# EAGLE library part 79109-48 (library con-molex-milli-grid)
RECEPTACAL
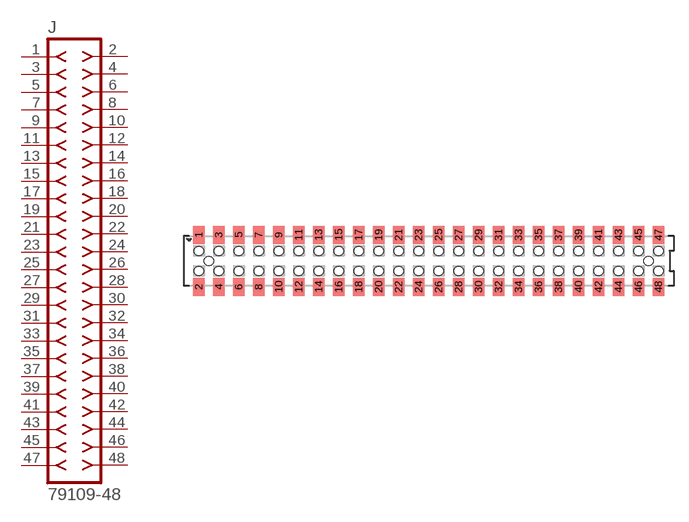
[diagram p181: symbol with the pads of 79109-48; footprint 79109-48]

Designator prefix J

## 79109-48  [79109-48]
1  1  pas
2  2  pas
3  3  pas
4  4  pas
5  5  pas
6  6  pas
7  7  pas
8  8  pas
9  9  pas
10  10  pas
11  11  pas
12  12  pas
13  13  pas
14  14  pas
15  15  pas
16  16  pas
17  17  pas
18  18  pas
19  19  pas
20  20  pas
21  21  pas
22  22  pas
23  23  pas
24  24  pas
25  25  pas
26  26  pas
27  27  pas
28  28  pas
29  29  pas
30  30  pas
31  31  pas
32  32  pas
33  33  pas
34  34  pas
35  35  pas
36  36  pas
37  37  pas
38  38  pas
39  39  pas
40  40  pas
41  41  pas
42  42  pas
43  43  pas
44  44  pas
45  45  pas
46  46  pas
47  47  pas
48  48  pas

## Footprint 79109-48 (pad centres in mm)
RECEPTACAL SMD Dual Row, Vertical, Pass-Thru
smd 1.12 x 1.83: 1 -23,2.6; 2 -23,-2.6; 3 -21,2.6; 4 -21,-2.6; 5 -19,2.6; 6 -19,-2.6; 7 -17,2.6; 8 -17,-2.6; 9 -15,2.6; 10 -15,-2.6; 11 -13,2.6; 12 -13,-2.6; 13 -11,2.6; 14 -11,-2.6; 15 -9,2.6; 16 -9,-2.6; 17 -7,2.6; 18 -7,-2.6; 19 -5,2.6; 20 -5,-2.6; 21 -3,2.6; 22 -3,-2.6; 23 -1,2.6; 24 -1,-2.6; 25 1,2.6; 26 1,-2.6; 27 3,2.6; 28 3,-2.6; 29 5,2.6; 30 5,-2.6; 31 7,2.6; 32 7,-2.6; 33 9,2.6; 34 9,-2.6; 35 11,2.6; 36 11,-2.6; 37 13,2.6; 38 13,-2.6; 39 15,2.6; 40 15,-2.6; 41 17,2.6; 42 17,-2.6; 43 19,2.6; 44 19,-2.6; 45 21,2.6; 46 21,-2.6; 47 23,2.6; 48 23,-2.6
hole 0.914 at -22,0
hole 0.914 at -23,1
hole 0.914 at -23,-1
hole 0.914 at -21,-1
hole 0.914 at -21,1
hole 0.914 at -19,-1
hole 0.914 at -19,1
hole 0.914 at -17,1
hole 0.914 at -17,-1
hole 0.914 at -15,1
hole 0.914 at -15,-1
hole 0.914 at -13,1
hole 0.914 at -13,-1
hole 0.914 at -11,1
hole 0.914 at -11,-1
hole 0.914 at -9,-1
hole 0.914 at -9,1
hole 0.914 at -7,1
hole 0.914 at -7,-1
hole 0.914 at -5,1
hole 0.914 at -5,-1
hole 0.914 at -3,1
hole 0.914 at -3,-1
hole 0.914 at -1,-1
hole 0.914 at -1,1
hole 0.914 at 1,1
hole 0.914 at 3,1
hole 0.914 at 5,1
hole 0.914 at 1,-1
hole 0.914 at 3,-1
hole 0.914 at 5,-1
hole 0.914 at 7,-1
hole 0.914 at 9,-1
hole 0.914 at 11,-1
hole 0.914 at 13,-1
hole 0.914 at 15,-1
hole 0.914 at 7,1
hole 0.914 at 9,1
hole 0.914 at 11,1
hole 0.914 at 13,1
hole 0.914 at 15,1
hole 0.914 at 17,-1
hole 0.914 at 19,-1
hole 0.914 at 17,1
hole 0.914 at 19,1
hole 0.914 at 21,1
hole 0.914 at 23,1
hole 0.914 at 21,-1
hole 0.914 at 23,-1
hole 0.914 at 22,0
